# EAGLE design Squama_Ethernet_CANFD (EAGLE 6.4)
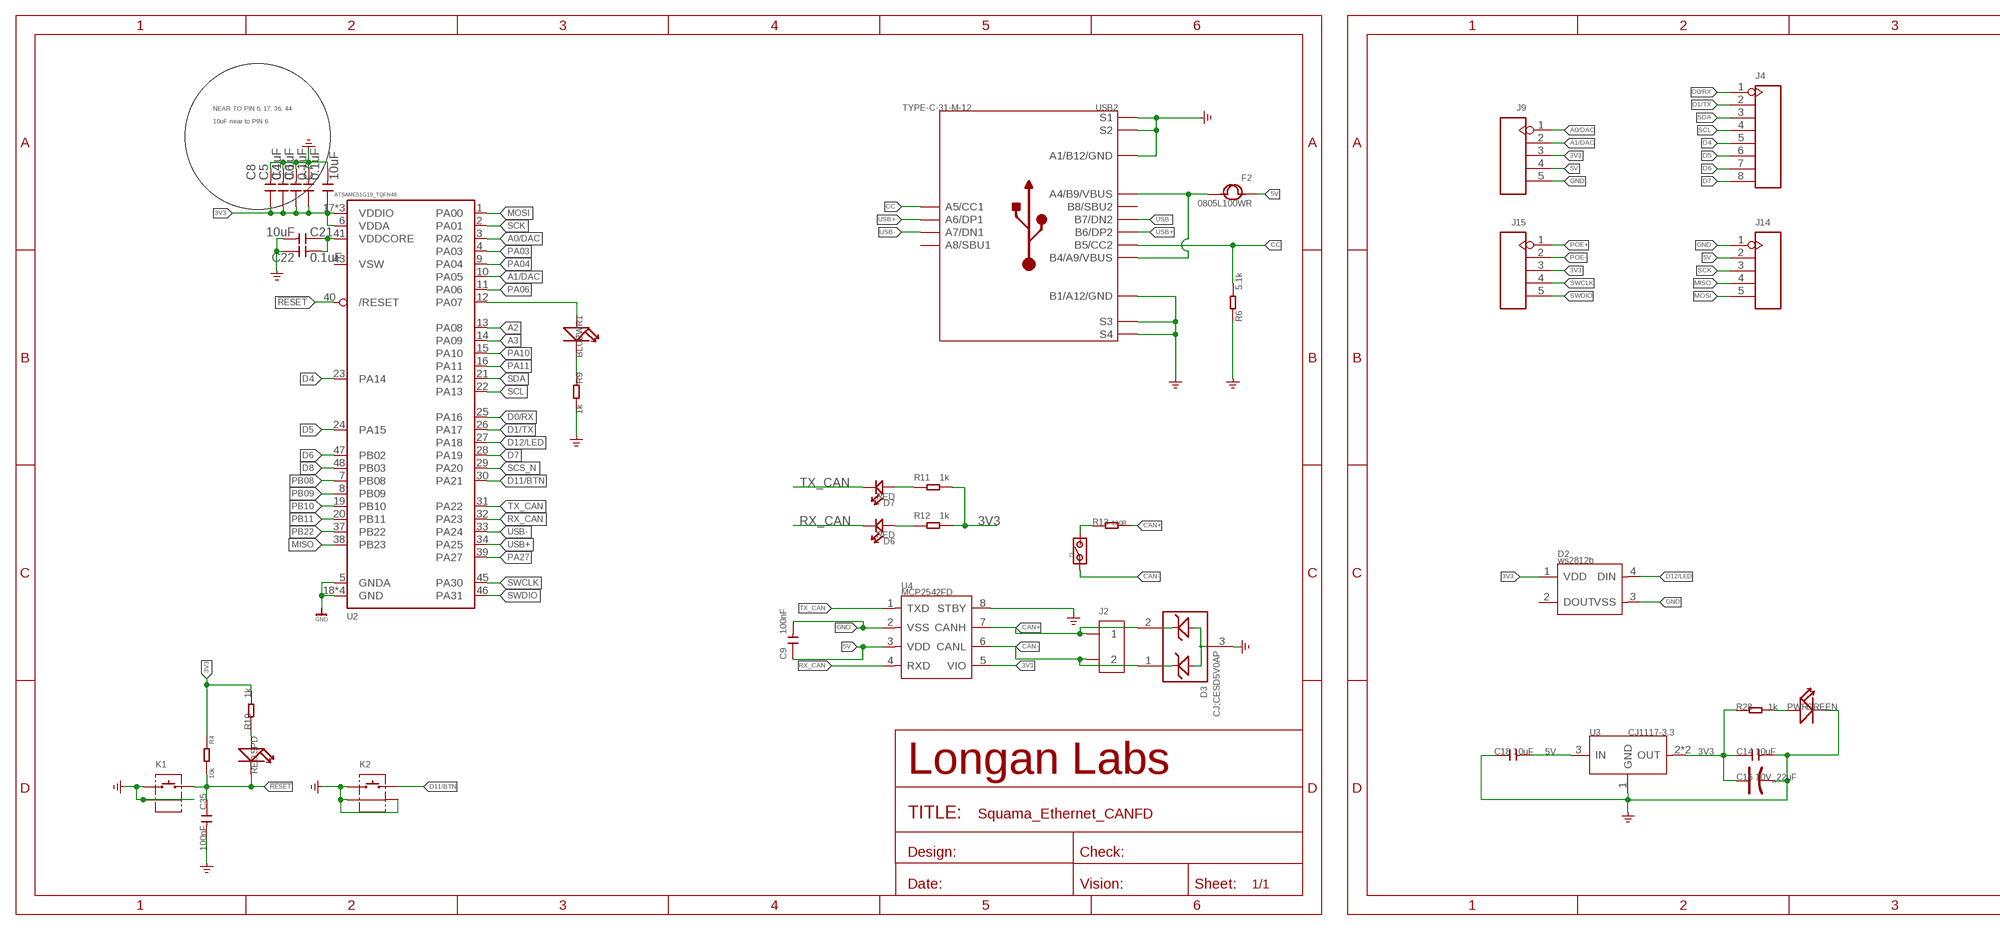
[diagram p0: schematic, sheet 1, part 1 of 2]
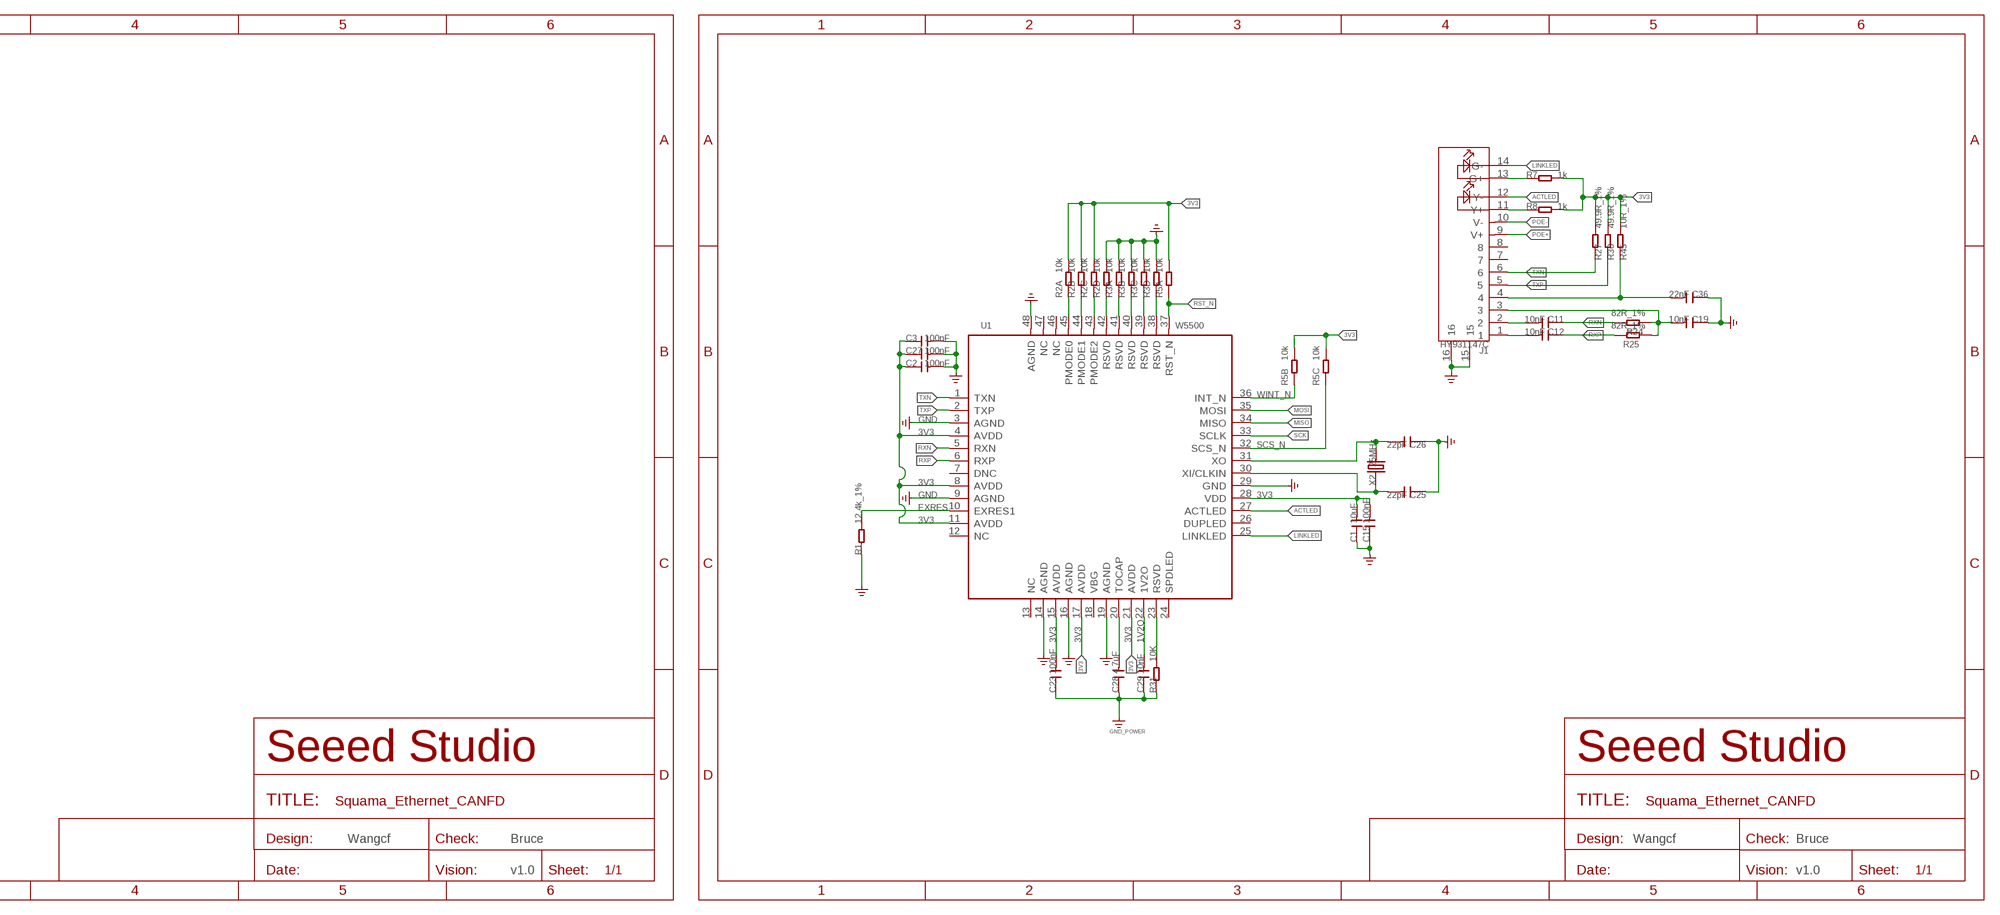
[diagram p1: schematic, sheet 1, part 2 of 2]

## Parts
C1  10uF  C-0603  [C0603]
C2  100nF  C-0603  [C0603]
C3  100nF  C-0603  [C0603]
C4  0.1uF  CAP-0603  [C0603]
C5  0.1uF  CAP-0603  [C0603]
C6  0.1uF  CAP-0603  [C0603]
C7  10uF  CAP-0603  [C0603]
C8  0.1uF  CAP-0603  [C0603]
C9  100nF  CAP-0603  [C0603]
C11  10nF  C-0603  [C0603]
C12  10nF  C-0603  [C0603]
C14  10uF  C-0805  [C0805]
C15  100nF  C-0603  [C0603]
C16  10V_22uF  CAP-AVX-B  [AVX-B]
C18  10uF  C-0805  [C0805]
C19  10nF  C-0603  [C0603]
C21  0.1uF  CAP-0603  [C0603]
C22  10uF  CAP-0603  [C0603]
C23  100nF  C-0603  [C0603]
C25  22pF  C-0603  [C0603]
C26  22pF  C-0603  [C0603]
C27  100nF  C-0603  [C0603]
C28  4.7uF  C-0805  [C0805]
C29  10nF  C-0603  [C0603]
C35  100nF  CAP-0603  [C0603]
C36  22nF  C-0603  [C0603]
D2  ws2812b  LED-RGB-4P-WS2812B-304990003  [LED4-SMD-5050]
D3  CJ;CESD5V0AP  D-ESD-3P'CESD3V3AP'  [SOT-23]
D6  RED  LED'0603'  [LED-0603]
D7  RED  LED'0603'  [LED-0603]
F2  0805L100WR  FUSE0805  [F0805]
J1  HY931147C  RJ45-HY931147C  [RJ45-14+2P-16.1X21.6X13.95MM]
J2  SCREW-TERMINAL-2P'3.5'  [H2-3.5-7.0X7.0MM]
J4  HEADER-8P-80/40MIL  [H8-2.54-C80D40MIL]
J9  HEADER-5P-2.54  [H5-2.54]
J14  HEADER-5P-2.0  [H5-2.0]
J15  HEADER-5P-2.0  [H5-2.0]
K1  BUTTON-2+2P  [SW2+2P-7.7X2.75X3.95MM]
K2  BUTTON-2+2P  [SW2+2P-7.7X2.75X3.95MM]
P1  PAD-JUMPER-2P  [2P-SMD-1.78X1.27]
PWR  GREEN  LED'0603'  [LED-0603]
PWR1  BLUE  LED'0603'  [LED-0603]
R1  12.4k_1%  R-0603  [0603]
R2  10k  RES-ARRAY-0804  [R0804-8]
R3  10k  RES-ARRAY-0804  [R0804-8]
R4  10k  RES-0603  [R0603]
R5  10k  RES-ARRAY-0804  [R0804-8]
R6  5.1k  RES-0603  [R0603]
R7  1k  R-0603  [0603]
R8  1k  R-0603  [0603]
R9  1k  R-0603  [0603]
R10  1k  R-0603  [0603]
R11  1k  RES-0603  [R0603]
R12  1k  RES-0603  [R0603]
R13  120R  R-0603  [0603]
R24  82R_1%  R-0603  [0603]
R25  82R_1%  R-0603  [0603]
R27  49.9R_1%  R-0603  [0603]
R28  1k  R-0603  [0603]
R30  49.9R_1%  R-0603  [0603]
R31  10K  R-0603  [0603]
R45  10R_1%  R-0603  [0603]
SPD  RED  LED'0603'  [LED-0603]
U1  W5500  DRIVER-W5500  [LQFP-48]
U2  ATSAME51G19_TQFN48  [TQFN48_7MM]
U3  CJ1117-3.3  PMIC-CJ1117'SOT89'  [SOT-89]
U4  MCP2542FD  TRANSCEIVER-MCP2542  [SOIC8-1.27-5X4MM]
USB2  TYPE-C-31-M-12  USB2.0-TYPE-C  [USB2.0-TYPE-C]
X2  25MHz  CRYSTAL'5032'  [2P-SMD-5X3.2]

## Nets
1V2O: C29.2 U1.22(1V2O)
3V3: C1.2 C2.1 C3.1 C4.1 C5.1 C6.1 C7.1 C8.1 C14.1 C15.2 C16.+ C23.2 C27.1 D2.1(VDD) J9.3 J15.3 R2.6 R2.7 R2.8 R4.1 R5.6 R5.7 R5.8 R7.2 R8.2 R10.2 R11.2 R12.2 R27.2 R28.1 R30.2 R45.2 U1.4(AVDD) U1.8(AVDD) U1.11(AVDD) U1.15(AVDD) U1.17(AVDD) U1.21(AVDD) U1.28(VDD) U2.6(VDDA) U2.17(VDDIO) U2.36(VDDIO) U2.44(VDDIO) U3.2(OUT) U3.4(OUT) U4.5(VIO)
5V [usbvcc]: C9.1 C18.2 F2.1 J9.4 J14.2 U3.3(IN) U4.3(VDD)
!RESET: C35.1 K1.2 R4.2 SPD.- U2.40(/RESET)
A0/DAC: J9.1 U2.3(PA02)
A1/DAC: J9.2 U2.10(PA05)
A2: U2.13(PA08)
A3: U2.14(PA09)
ACTLED: J1.12(Y-) U1.27(ACTLED)
CAN+: D3.2 J2.1 R13.2 U4.7(CANH)
CAN-: D3.1 J2.2 P1.1 U4.6(CANL)
CC: R6.2 USB2.A5(A5/CC1) USB2.B5(B5/CC2)
D0/RX: J4.1 U2.25(PA16)
D1/TX: J4.2 U2.26(PA17)
D4: J4.5 U2.23(PA14)
D5: J4.6 U2.24(PA15)
D6: J4.7 U2.47(PB02)
D7: J4.8 U2.28(PA19)
D8: U2.48(PB03)
D11/BTN: K2.2 U2.30(PA21)
D12/LED: D2.4(DIN) U2.27(PA18)
EXRES: R1.2 U1.10(EXRES1)
GND: C1.1 C2.2 C3.2 C4.2 C5.2 C6.2 C7.2 C8.2 C9.2 C14.2 C15.1 C16.- C18.1 C19.1 C21.1 C22.2 C23.1 C25.1 C26.1 C27.2 C28.1 C29.1 C35.2 C36.1 D2.3(VSS) D3.3 J1.15 J1.16 J9.5 J14.1 K1.1 K1.S1 K1.S2 K2.1 K2.S1 K2.S2 PWR.- R1.1 R2.5 R3.5 R3.6 R3.7 R3.8 R6.1 R9.2 R31.1 U1.3(AGND) U1.9(AGND) U1.14(AGND) U1.16(AGND) U1.19(AGND) U1.29(GND) U1.48(AGND) U2.5(GNDA) U2.18(GND) U2.35(GND) U2.42(GND) U2.THERMAL(GND) U3.1(GND) U4.2(VSS) U4.8(STBY) USB2.A1_B12(A1/B12/GND) USB2.B1_A12(B1/A12/GND) USB2.S1 USB2.S2 USB2.S3 USB2.S4 USB2.S5(S1) USB2.S6(S2) ; supply symbol labelled GND_POWER
LINKLED: J1.14(G-) U1.25(LINKLED)
MISO: J14.4 U1.34(MISO) U2.38(PB23)
MOSI: J14.5 U1.35(MOSI) U2.1(PA00)
N$1: C25.2 U1.30(XI/CLKIN) X2.1
N$2: PWR1.- R9.1
N$3: F2.2 USB2.A4_B9(A4/B9/VBUS) USB2.B4_A9(B4/A9/VBUS)
N$4: J1.13(G+) R7.1
N$5: J1.11(Y+) R8.1
N$6: R10.1 SPD.+
N$7: PWR1.+ U2.12(PA07)
N$8: D7.+ R11.1
N$9: C21.2 C22.1 U2.41(VDDCORE)
N$10: P1.2 R13.1
N$15: D6.+ R12.1
N$16: C36.2 J1.4 R45.1
N$23: C11.2 J1.2
N$24: C12.2 J1.1
N$26: PWR.+ R28.2
N$27: R3.4 U1.38(RSVD)
N$30: R3.3 U1.39(RSVD)
N$31: R3.2 U1.40(RSVD)
N$32: R3.1 U1.41(RSVD)
N$33: R2.4 U1.42(RSVD)
N$34: C19.2 J1.3 R24.2 R25.1
N$35: R2.3 U1.43(PMODE2)
N$36: R2.2 U1.44(PMODE1)
N$37: R2.1 U1.45(PMODE0)
N$50: R31.2 U1.23(RSVD)
PA03: U2.4(PA03)
PA04: U2.9(PA04)
PA06: U2.11(PA06)
PA10: U2.15(PA10)
PA11: U2.16(PA11)
PA27: U2.39(PA27)
PB08: U2.7(PB08)
PB09: U2.8(PB09)
PB10: U2.19(PB10)
PB11: U2.20(PB11)
PB22: U2.37(PB22)
POE+: J1.9(V+) J15.1
POE-: J1.10(V-) J15.2
RST_N: R5.1 U1.37(RST_N)
RX_CAN: D6.- U2.32(PA23) U4.4(RXD)
RXN: C11.1 R24.1 U1.5(RXN)
RXP: C12.1 R25.2 U1.6(RXP)
SCK: J14.3 U1.33(SCLK) U2.2(PA01)
SCL: J4.4 U2.22(PA13)
SCS_N: R5.3 U1.32(SCS_N) U2.29(PA20)
SDA: J4.3 U2.21(PA12)
SWCLK: J15.4 U2.45(PA30)
SWDIO: J15.5 U2.46(PA31)
TOCAP: C28.2 U1.20(TOCAP)
TX_CAN: D7.- U2.31(PA22) U4.1(TXD)
TXN: J1.6 R27.1 U1.1(TXN)
TXP: J1.5 R30.1 U1.2(TXP)
USB+: U2.34(PA25) USB2.A6(A6/DP1) USB2.B6(B6/DP2)
USB-: U2.33(PA24) USB2.A7(A7/DN1) USB2.B7(B7/DN2)
WINT_N: R5.2 U1.36(INT_N)
XO: C26.2 U1.31(XO) X2.2
Unconnected: D2.2(DOUT) J1.7 J1.8 R5.4 R5.5 U1.7(DNC) U1.12(NC) U1.13(NC) U1.18(VBG) U1.24(SPDLED) U1.26(DUPLED) U1.46(NC) U1.47(NC) U2.43(VSW) USB2.A8(A8/SBU1) USB2.B8(B8/SBU2)

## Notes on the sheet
- NEAR TO PIN 6, 17, 36, 44
- 10uF near to PIN 6
- Wangcf | Bruce | Wangcf | Bruce
- v1.0 | v1.0

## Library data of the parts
C1-C3 C11 C12 C14 C15 C18 C19 C23 C25-C29 C36 = Discrete:C*: Ceramic Capacitors
C4-C9 C21 C22 C35 = Discrete-new:CAP: Ceramic Capacitors
C16 = Discrete:CAP*: Electrolytic Capacitors,Tantalum Capacitors and Super Capacitors
D2 = Discrete-new:LED-RGB-4P
D3 = Discrete-new:D-ESD-3P: 304060003
D6 D7 = Discrete-new:LED
F2 = Discrete-small:FUSE
J1 = Connector-new:RJ45-HY931147C
J2 = Connector-new:SCREW-TERMINAL-2P: 2P-3.5:320110028;2P-5.0:320110031
J4 = Connector-new:HEADER-8P
J9 J14 J15 = Connector-new:HEADER-5P
K1 K2 = Connector-new:BUTTON-2+2P
P1 = Discrete:PAD-JUMPER-2P
PWR PWR1 SPD = Discrete:LED*
R1 R7-R10 R13 R24 R25 R27 R28 R30 R31 R45 = Discrete:R*
R2 R3 R5 = Discrete-new:RES-ARRAY: Resistor Array
R4 R6 R11 R12 = Discrete-new:RES
U1 = template:DRIVER-W5500
U2 = MyLibrary:ATSAME51G19; MPN: ATSAME51G19A-MF
U3 = IC-new:PMIC-CJ*1117: Low Drop Fixed And Adjustable Positive Voltage Regulators http://www.datasheetcatalog.org/datasheet/SGSThomsonMicroelectronics/mXuqtqv.pdf
U4 = untitled:TRANSCEIVER-MCP2542
USB2 = Connector-new:USB2.0-TYPE-C
X2 = Discrete:CRYSTAL*: CRYSTAL

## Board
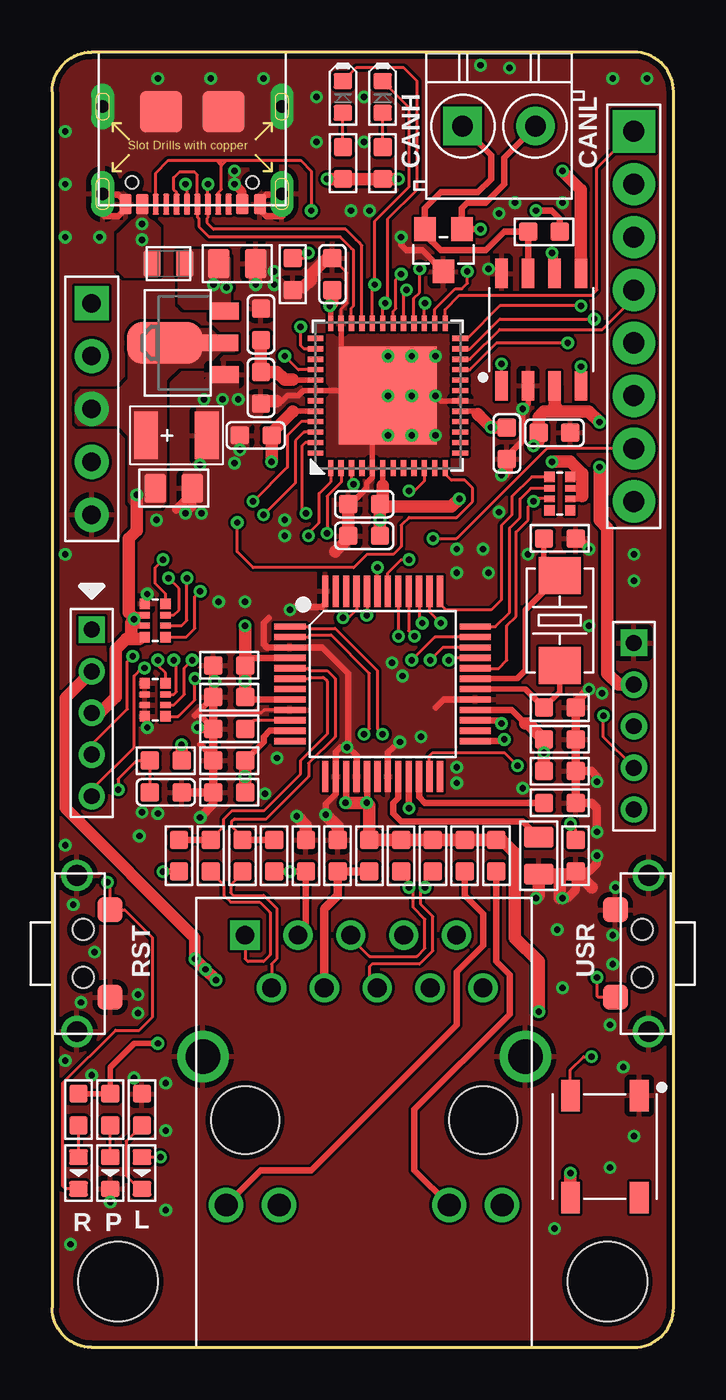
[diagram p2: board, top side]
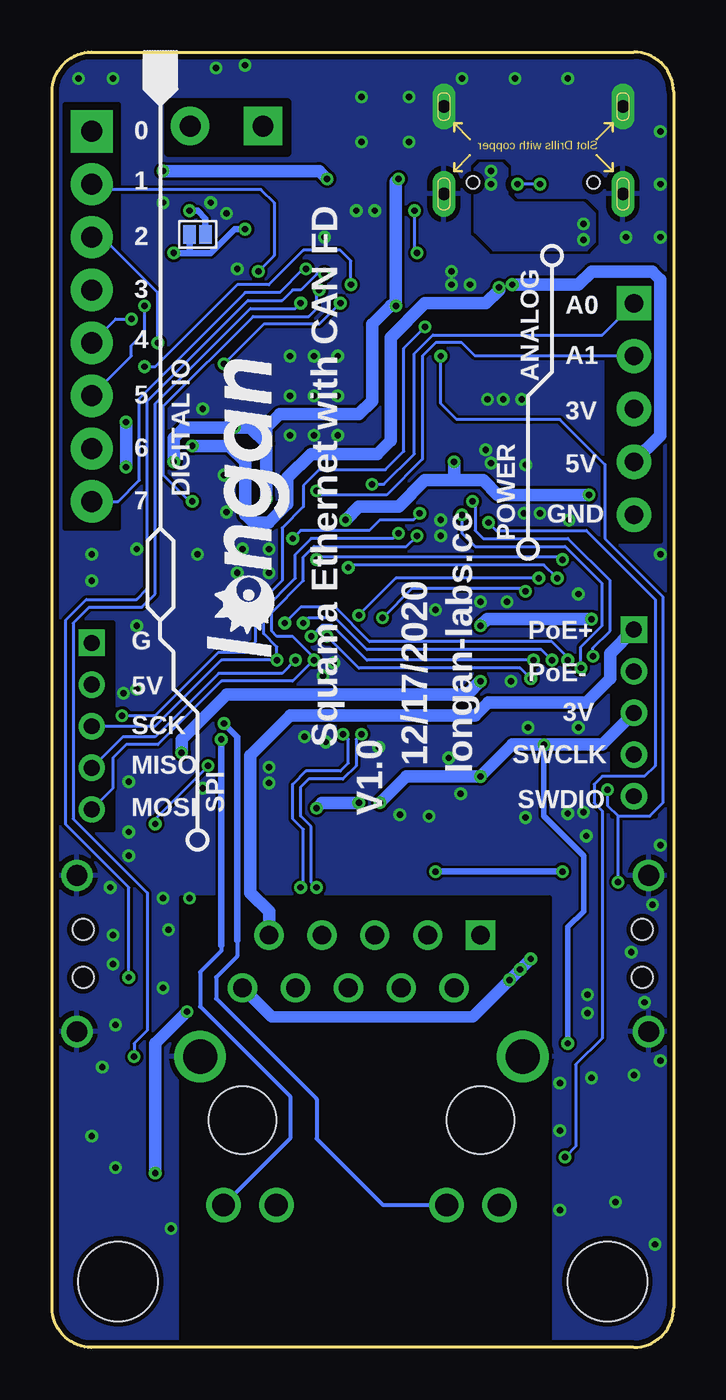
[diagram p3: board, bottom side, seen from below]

Size 29.84 x 62.23 mm. Coordinates in mm from the lower left corner, seen from the top.
Outline: 1.91,0 27.94,0 arc90 29.84,1.91 29.84,60.33 arc90 27.94,62.23 1.91,62.23 arc90 0,60.33 0,1.91 arc90 1.91,0
Copper layers (1*16): Top 0.035mm / dielectric 1.5mm / Bottom 0.035mm
Design rules "default *": minimum track width 5mil, minimum drill 12mil, track to track 4mil, track to pad 4mil, pad to pad 4mil, via to via 4mil, smd to smd 0mil, copper to edge 10mil, drill to drill 10mil, minimum pad ring 10mil, minimum via ring 6mil, stop-mask expansion 2mil, vias tented up to drill 25mil, thermal gap 10mil
Holes 3.81 mm at 26.67,3.17 3.17,3.17
bRestrict: area 0.6,38.7 to 3.2,51.4; area 0.9,25.5 to 2.9,35.4; area 26.7,39.4 to 29.2,59.7; area 26.9,24.9 to 29,34.8; area 6,0 to 23.6,21.6; area 0.6,38.7 to 3.2,51.4; area 18.5,57.4 to 24.3,59.8

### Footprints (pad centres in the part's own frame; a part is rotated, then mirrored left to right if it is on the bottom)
C0603 = smd 0.889 x 0.889: 1 -0.762,0; 2 0.762,0
C0805 = smd 1.016 x 1.397: 1 -0.889,0; 2 0.889,0
AVX-B = smd 1.143 x 2.286: + -1.46,0; - 1.46,0
LED4-SMD-5050 = smd 0.9 x 1.5: 1 -1.65,-2.45; 2 1.65,-2.45; 3 1.65,2.45; 4 -1.65,2.45
SOT-23 = smd 1.016 x 1.143: 1 -0.889,-1.016; 2 0.889,-1.016; 3 0,1.016
LED-0603 = smd 0.762 x 0.889: + 0.762,0; - -0.762,0
F0805 = smd 0.819 x 1.27: 1 -0.79,0; 2 0.79,0
RJ45-14+2P-16.1X21.6X13.95MM = drill 0.9 pad 1.4 square: 1 5.72,-8.89 | drill 0.9 pad 1.4: 2 4.45,-6.35; 3 3.18,-8.89; 4 1.91,-6.35; 5 0.64,-8.89; 6 -0.63,-6.35; 7 -1.9,-8.89; 8 -3.17,-6.35; 9 -4.44,-8.89; 10 -5.71,-6.35 | drill 1.1 pad 1.6: 11 6.625,4.08; 12 4.085,4.08; 13 -4.085,4.08; 14 -6.625,4.08 | drill 1.65 pad 2.3: 15 7.745,-3.05; 16 -7.745,-3.05 | hole 3.25: -5.715,0; 5.715,0
H2-3.5-7.0X7.0MM = drill 1 pad 1.85 square: 1 -1.75,0 | drill 1 pad 1.85: 2 1.75,0
H8-2.54-C80D40MIL = drill 1.016 pad 2.032 square: 1 0,8.89 | drill 1.016 pad 2.032: 2 0,6.35; 3 0,3.81; 4 0,1.27; 5 0,-1.27; 6 0,-3.81; 7 0,-6.35; 8 0,-8.89
H5-2.54 = drill 0.889 pad 1.651 square: 1 0,5.08 | drill 0.889 pad 1.651: 2 0,2.54; 3 0,0; 4 0,-2.54; 5 0,-5.08
H5-2.0 = drill 0.762 pad 1.27 square: 1 0,4 | drill 0.762 pad 1.27: 2 0,2; 3 0,0; 4 0,-2; 5 0,-4
SW2+2P-7.7X2.75X3.95MM = smd 1.2 x 1.2: 1 -2.1,0; 2 2.1,0 | drill 1 pad 1.5: S1 -3.75,1.6; S2 3.75,1.6 | hole 1: -1.15,1.3; 1.15,1.3
2P-SMD-1.78X1.27 = smd 0.889 x 0.61: 1 0,0.381; 2 0,-0.381
LED-0603' = smd 0.762 x 0.889: + -0.762,0; - 0.762,0
0603 = smd 0.889 x 0.889: 1 -0.762,0; 2 0.762,0
R0804-8 = smd 0.498 x 0.5: 1 -0.801,-0.5; 4 0.801,-0.5; 5 0.801,0.5; 8 -0.801,0.5 | smd 0.3 x 0.5: 2 -0.25,-0.5; 3 0.25,-0.5; 6 0.25,0.5; 7 -0.25,0.5
R0603 = smd 0.889 x 0.889: 1 -0.762,0; 2 0.762,0
LQFP-48 = smd 1.5 x 0.3: 1 -4.45,2.75; 2 -4.45,2.25; 3 -4.45,1.75; 4 -4.45,1.25; 5 -4.45,0.75; 6 -4.45,0.25; 7 -4.45,-0.25; 8 -4.45,-0.75; 9 -4.45,-1.25; 10 -4.45,-1.75; 11 -4.45,-2.25; 12 -4.45,-2.75; 25 4.45,-2.75; 26 4.45,-2.25; 27 4.45,-1.75; 28 4.45,-1.25; 29 4.45,-0.75; 30 4.45,-0.25; 31 4.45,0.25; 32 4.45,0.75; 33 4.45,1.25; 34 4.45,1.75; 35 4.45,2.25; 36 4.45,2.75 | smd 0.3 x 1.5: 13 -2.75,-4.45; 14 -2.25,-4.45; 15 -1.75,-4.45; 16 -1.25,-4.45; 17 -0.75,-4.45; 18 -0.25,-4.45; 19 0.25,-4.45; 20 0.75,-4.45; 21 1.25,-4.45; 22 1.75,-4.45; 23 2.25,-4.45; 24 2.75,-4.45; 37 2.75,4.45; 38 2.25,4.45; 39 1.75,4.45; 40 1.25,4.45; 41 0.75,4.45; 42 0.25,4.45; 43 -0.25,4.45; 44 -0.75,4.45; 45 -1.25,4.45; 46 -1.75,4.45; 47 -2.25,4.45; 48 -2.75,4.45
TQFN48_7MM = smd 0.25 x 0.75: 1 -2.75,-3.475; 2 -2.25,-3.475; 3 -1.75,-3.475; 4 -1.25,-3.475; 5 -0.75,-3.475; 6 -0.25,-3.475; 7 0.25,-3.475; 8 0.75,-3.475; 9 1.25,-3.475; 10 1.75,-3.475; 11 2.25,-3.475; 12 2.75,-3.475; 25 2.75,3.475; 26 2.25,3.475; 27 1.75,3.475; 28 1.25,3.475; 29 0.75,3.475; 30 0.25,3.475; 31 -0.25,3.475; 32 -0.75,3.475; 33 -1.25,3.475; 34 -1.75,3.475; 35 -2.25,3.475; 36 -2.75,3.475 | smd 0.75 x 0.25: 13 3.475,-2.75; 14 3.475,-2.25; 15 3.475,-1.75; 16 3.475,-1.25; 17 3.475,-0.75; 18 3.475,-0.25; 19 3.475,0.25; 20 3.475,0.75; 21 3.475,1.25; 22 3.475,1.75; 23 3.475,2.25; 24 3.475,2.75; 37 -3.475,2.75; 38 -3.475,2.25; 39 -3.475,1.75; 40 -3.475,1.25; 41 -3.475,0.75; 42 -3.475,0.25; 43 -3.475,-0.25; 44 -3.475,-0.75; 45 -3.475,-1.25; 46 -3.475,-1.75; 47 -3.475,-2.25; 48 -3.475,-2.75 | smd 4.7 x 4.7: THERMAL 0,0
SOT-89 = smd 0.8 x 1.4: 1 -1.524,-1.905; 3 1.524,-1.905 | smd 0.8 x 1.9: 2 0,-1.651 | smd 2.032 x 3.65: 4 0,0.94
SOIC8-1.27-5X4MM = smd 0.6 x 1.4: 1 -1.905,-2.7; 2 -0.635,-2.7; 3 0.635,-2.7; 4 1.905,-2.7; 5 1.905,2.7; 6 0.635,2.7; 7 -0.635,2.7; 8 -1.905,2.7
USB2.0-TYPE-C = smd 1 x 0.6: A1_B12 -0.05,3.25; A4_B9 -0.05,2.4; B1_A12 -0.05,-3.2; B4_A9 -0.05,-2.4 | smd 1 x 0.3: A5 -0.05,1.25; A6 -0.05,0.25; A7 -0.05,-0.25; A8 -0.05,-1.25; B5 -0.05,-1.75; B6 -0.05,-0.75; B7 -0.05,0.75; B8 -0.05,1.75 | drill 0.6 pad 1 long: S1 -4.75,4.3; S2 -4.75,-4.3 | drill 0.6 pad 1.1 long: S3 -0.55,4.3; S4 -0.55,-4.3 | smd 2 x 2: S5 -4.5,1.5; S6 -4.5,-1.5 | hole 0.6: -1.1,-2.89; -1.1,2.89
2P-SMD-5X3.2 = smd 1.778 x 2.032: 1 -2.159,0; 2 2.159,0

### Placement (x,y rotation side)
C1  24.38,27.69 180 top
C2  8.51,28.19 180 top
C3  8.51,32.77 180 top
C4  13.46,51.56 90 top
C5  9.78,43.81 180 top
C6  21.84,43.43 270 top
C7  14.99,38.99 180 top
C8  14.99,40.51 180 top
C9  24.13,43.94 0 top
C11  9.14,23.62 270 top
C12  7.62,23.62 270 top
C14  5.84,41.27 0 top
C15  24.38,29.21 180 top
C16  5.97,43.81 0 top
C18  8.89,52.07 180 top
C19  12.19,23.62 270 top
C21  10.03,49.15 270 top
C22  10.03,46.1 270 top
C23  8.51,26.67 0 top
C25  24.38,30.73 180 top
C26  24.38,38.86 180 top
C27  8.51,31.24 180 top
C28  23.37,23.62 90 top
C29  24.38,26.16 180 top
C35  5.46,26.67 0 top
C36  13.72,23.62 270 top
D2  26.54,9.65 0 top
D3  18.8,52.7 180 top
D6  15.88,60.07 270 top
D7  13.97,60.07 270 top
F2  5.59,52.07 180 top
J1  14.99,10.92 180 top
J2  21.46,58.67 0 top
J4  27.94,49.53 0 top
J9  1.91,45.09 0 top
J14  27.94,29.84 0 top
J15  1.91,30.48 0 top
K1  2.79,18.92 90 top
K2  27.05,18.92 270 top
P1  22.86,53.47 90 bottom
PWR  GREEN  [LED-0603']  2.79,8.38 270 top
PWR1  BLUE  [LED-0603']  4.32,8.38 270 top
R1  8.51,29.72 0 top
R2  4.95,34.92 90 top
R3  4.95,31.11 90 top
R4  5.46,28.19 180 top
R5  24.38,41.02 270 top
R6  11.56,51.56 90 top
R7  21.34,23.62 90 top
R8  19.81,23.62 90 top
R9  4.32,11.43 90 top
R10  1.27,11.43 90 top
R11  13.97,56.9 270 top
R12  15.88,56.9 270 top
R13  23.62,53.59 180 top
R24  10.67,23.62 270 top
R25  6.1,23.62 90 top
R27  18.29,23.62 90 top
R28  2.79,11.43 270 top
R30  16.76,23.62 90 top
R31  25.15,23.62 90 top
R45  15.24,23.62 90 top
SPD  RED  [LED-0603']  1.27,8.38 270 top
U1  15.88,31.88 0 top
U2  16.13,45.72 0 top
U3  6.35,48.26 90 top
U4  23.5,48.9 0 top
U$7  [LONGAN-SILK-SMALLER]  17.27,31.88 90 bottom
USB2  6.73,54.86 270 top
X2  24.38,34.92 90 top

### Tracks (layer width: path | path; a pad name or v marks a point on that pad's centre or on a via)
1V2O
  Top 0.305: U1.22 17.62,26.44 17.91,26.16 C29.2
3V3  (via drill 0.3 pad 0.51, 0.3 pad 0.61)
  Top 0.254: R10.2 2.67,12.19 2.79,12.06 R28.1 2.79,13.46 3.94,14.61 v5.08,14.61 | U2.36 13.38,49.99 v13.34,50.04 | U2.6 15.88,41.41 15.88,41.4 | U2.44 11.57,44.97 11.56,44.96 | U2.17 20.31,44.97 20.51,44.77
  Top 0.305: U1.15 14.12,26.19 v14.1,26.16 | U1.17 15.12,26.17 v15.11,26.16 | U1.21 17.12,25.93 v17.14,25.91 | U1.28 22.08,30.63 22.73,29.97 | U1.8 9.39,31.13 C27.1 | U1.11 10.45,29.63 10.16,29.34 10.16,29.08 C2.1 | U1.4 9.63,33.13 C3.1 | R2.7 4.12,34.67 3.94,34.86 3.94,34.92 v3.94,34.99 4.12,35.17 R2.6 | R5.7 25.46,41.27 | R5.6 25.34,40.77 25.46,40.89 | R5.8 25.42,41.82 25.46,41.78
  Top 0.406: R2.8 4.28,34.12 4.19,34.04
  Top 0.61: C23.2 v9.27,27.43 C2.1 | v14.1,26.16 v15.11,26.16 15.24,26.04 R45.2 R30.2 R27.2 R8.2 R7.2 21.59,24.38 22.23,23.75 22.23,19.68 23.37,18.54 v23.37,16.13 | 22.73,29.97 22.86,29.97 C15.2 v23.62,28.57 C1.2 | C27.1 v9.27,32 C3.1 v9.27,34.67 | R4.1 v6.22,28.96 | J15.3 2.29,30.48 3.05,31.24 3.05,33.53 3.56,34.04 3.81,34.04 | 3.81,34.04 4.19,34.04 | 3.81,34.04 3.81,34.8 3.94,34.92 | v3.94,34.99 3.94,35.05 3.68,35.31 3.68,38.86 4.06,39.24 v4.06,40.96 | 25.46,40.89 25.46,41.27 25.46,41.78 25.46,41.97 24.89,42.55 v24,42.55 | D2.1 v24.89,8.38 | C4.1 13.46,50.16 v13.34,50.04 | 15.88,41.4 15.88,40.64 C8.1 15.75,40.39 | 15.75,40.39 v15.75,39.75 C7.1 | v10.54,42.55 C5.1 10.54,43.94 11.56,44.96 | C6.1 v21.08,44.2 20.51,44.77 20.45,44.83 | 15.75,40.39 19.18,40.39 v19.56,40.77 | v13.21,56.13 R11.2 R12.2 v16.64,56.13 | U4.5 25.4,55.63 v24.51,56.52
  Bottom 0.254: v5.08,14.61 5.08,20.19 4.32,20.95 4.32,23.62 6.22,25.53 v6.22,28.96
  Bottom 0.61: v14.1,26.16 12.83,27.43 v9.27,27.43 7.75,28.96 v6.22,28.96 3.43,28.96 J15.3 | v15.11,26.16 16.89,26.16 v17.14,25.91 | v23.62,28.57 C15.2 21.46,31.37 9.91,31.37 v9.27,32 | v3.94,34.99 8.95,34.99 v9.27,34.67 | v24.89,8.38 24.89,14.61 v23.37,16.13 | v4.06,40.96 8.45,40.96 9.14,41.66 10.41,41.66 | v15.75,39.75 15.11,40.39 13.21,40.39 11.94,41.66 10.41,41.66 | v10.54,42.55 10.54,41.78 10.41,41.66 | v24,42.55 24,43.69 23.5,44.2 v21.08,44.2 20.32,44.2 | v19.56,40.77 19.56,43.43 | 19.56,43.43 19.56,44.2 | 20.32,44.2 19.56,44.2 | 19.56,43.43 20.32,44.2 | v13.21,56.13 13.34,56.01 v13.34,50.04 13.59,50.04 14.48,49.15 14.48,45.47 15.11,44.83 18.92,44.83 19.56,44.2 | v24.51,56.52 17.02,56.52 v16.64,56.13
  pour Top (isolate 0.254, no thermals): 7.62,48.9 4.19,48.9 3.68,48.39 3.68,46.48 3.17,45.97 1.4,45.97 1.14,45.72 1.14,44.45 1.27,44.32 3.17,44.32 3.68,43.81 3.68,40.64 3.94,40.39 5.21,40.39 5.46,40.64 5.46,46.48 6.1,47.12 7.37,47.12 8.13,47.88 8.76,47.88 8.76,48.51 8,48.51
5V  (via drill 0.3 pad 0.61)
  Top 0.61: J14.2 27.21,31.84 26.67,32.38 26.67,39.37 26.29,39.75 v26.29,42.29 | U4.3 24.13,45.21 | 24.13,45.21 23.88,44.96 | 24.38,44.96 24.13,44.96 23.88,44.96 | 24.13,45.21 24.38,44.96 | 23.88,44.96 23.62,44.96 23.37,44.7 C9.1 23.37,43.56 v23.11,43.31 | 24.38,44.96 25.78,44.96 v26.29,44.45
  Bottom 0.61: v7.75,51.05 4.57,51.05 3.94,51.69 1.02,51.69 0.64,51.31 0.64,43.81 J9.4 | v8.38,50.93 8.38,50.8 9.02,50.16 11.94,50.16 13.59,48.51 13.59,43.56 14.22,42.93 17.4,42.93 18.54,41.78 18.54,40.51 19.43,39.62 20.19,39.62 20.57,40.01 20.57,42.55 21.34,43.31 v23.11,43.31 | v26.29,42.29 v26.29,44.45
  pour Top (isolate 0.254, no thermals): 6.35,52.7 8,52.7 8.51,52.32 8.51,49.53 8.26,49.53 7.87,49.91 6.35,49.91 6.1,50.16 6.1,52.45
!RESET  (via drill 0.3 pad 0.61)
  Top 0.152: C35.1 R4.2 4.06,28.19 3.17,27.3 v3.17,26.8 | SPD.- 0.64,7.62 0.51,7.75 0.51,12.7 3.05,15.24 4.19,15.24 4.83,15.88 4.83,19.68 3.49,21.02 K1.2 2.79,22.23 v2.67,22.35 | U2.40 11.83,46.97 v11.18,47.62
  Bottom 0.152: v3.17,26.8 3.17,26.04 2.67,25.53 | 2.67,25.53 1.14,25.53 0.51,26.16 0.51,36.07 3.3,38.86 3.3,42.42 5.46,44.58 10.41,44.58 11.18,45.34 v11.18,47.62 | v2.67,22.35 2.67,25.53
A0/DAC  (via drill 0.3 pad 0.61)
  Top 0.152: U2.3 14.38,41.56 v14.48,41.47
  Bottom 0.152: v14.48,41.47 13.91,41.47 12.45,42.93 12.45,47.75 11.56,48.64 3.43,48.64 J9.1
A1/DAC  (via drill 0.3 pad 0.61)
  Top 0.152: U2.10 17.88,41.63 17.4,41.15 v17.14,41.15
  Bottom 0.152: J9.2 9.53,47.62 10.16,48.26 11.43,48.26 12.06,47.62 12.06,42.67 13.78,40.96 16.95,40.96 v17.14,41.15
ACTLED  (via drill 0.3 pad 0.61)
  Top 0.305: U1.27 21.43,30.13 v21.59,29.97
  Bottom 0.203: 20.95,19.56 20.95,18.8 21.97,17.78 21.97,16.76 17.14,11.94 17.14,10.03 13.97,6.86 10.92,6.86 J1.12
  Bottom 0.305: 20.95,19.56 20.95,29.34 v21.59,29.97
CAN+
  Top 0.305: U4.7 R13.2 21.72,53.59 20.83,52.7 18.67,52.7 17.91,53.47 D3.2 17.91,54.74 18.67,55.5 20.45,55.5 21.08,56.13 21.08,57.28 19.71,58.65 J2.1
CAN-  (via drill 0.3 pad 0.51)
  Top 0.305: U4.6 24.13,52.45 v24,52.58 | v20.57,53.72 D3.1 19.68,54.74 19.94,54.99 20.83,54.99 21.72,55.88 21.72,57.15 23.21,58.65 J2.2
  Bottom 0.305: v20.57,53.72 21.08,53.72 22.23,52.58 23.24,52.58 | 23.24,52.58 v24,52.58 | P1.1 23.24,52.58
CC  (via drill 0.3 pad 0.61)
  Top 0.152: USB2.A5 7.98,55.48 8.13,55.63 8.13,56.77 | USB2.B5 4.98,56.42 5.59,57.02 7.87,57.02 | 8.13,56.77 8.13,57.02 | 7.87,57.02 8.13,57.02 | 8.13,57.02 8.38,57.02 | 8.38,57.02 11.94,57.02 12.45,56.52 v12.45,54.61 | 8.13,56.77 7.87,57.02 | 8.38,57.02 8.13,56.77 | R6.2 12.06,52.32 v12.32,52.58
  Bottom 0.152: v12.45,54.61 12.45,52.7 v12.32,52.58
D0/RX
  Top 0.152: U2.25 18.88,49.87 19.56,50.55 25.91,50.55 26.16,50.8 26.16,56.64 J4.1
D1/TX  (via drill 0.3 pad 0.51)
  Top 0.152: U2.26 18.38,49.88 19.37,50.86 19.68,50.86 19.94,51.12 v19.94,51.69
  Bottom 0.152: J4.2 27.69,55.63 19.81,55.63 19.18,54.99 19.18,52.45 v19.94,51.69
D4  (via drill 0.3 pad 0.61)
  Top 0.152: U2.23 20.07,47.97 21.5,49.4 v26.04,49.4
  Bottom 0.152: J4.5 26.8,49.4 v26.04,49.4
D5  (via drill 0.3 pad 0.61)
  Top 0.152: U2.24 19.94,48.47 21.51,50.04 v25.4,50.04
  Bottom 0.152: J4.6 26.04,47.62 26.04,48.13 25.4,48.77 v25.4,50.04
D6  (via drill 0.3 pad 0.61)
  Top 0.152: U2.47 12.16,43.47 12,43.31 12,40.26 v12.19,40.07 | J4.7 23.75,43.18 19.43,38.86 v18.29,38.86
  Bottom 0.152: v12.19,40.07 12.51,39.75 14.1,39.75 14.61,39.24 17.91,39.24 v18.29,38.86
D7  (via drill 0.3 pad 0.51)
  Top 0.152: U2.28 17.38,50.4 17.65,50.67 v17.65,51.82
  Bottom 0.152: J4.8 26.67,40.64 25.65,41.66 25.65,45.59 20.57,50.67 18.92,50.67 17.78,51.82 v17.65,51.82
D11/BTN  (via drill 0.3 pad 0.51, 0.3 pad 0.61)
  Top 0.152: K2.2 26.22,16.82 26.16,16.88 v26.16,17.78 | U2.30 16.38,49.78 16.51,49.91 16.51,51.31 v16.76,51.56
  Bottom 0.152: v26.16,17.78 26.16,22.1 29.21,25.15 29.21,34.92 28.19,35.94 25.78,35.94 25.27,36.45 25.27,45.47 20.45,50.29 18.8,50.29 18.29,50.8 17.91,50.8 17.14,51.56 v16.76,51.56
D12/LED  (via drill 0.3 pad 0.51, 0.3 pad 0.61)
  Top 0.152: D2.4 24.89,13.34 25.53,13.97 v25.91,13.97 | U2.27 17.88,50.14 v17.91,50.16
  Bottom 0.152: v25.91,13.97 25.91,14.61 25.27,15.24 25.27,21.84 28.83,25.4 28.83,34.8 28.07,35.56 25.53,35.56 24.89,36.2 24.89,45.34 20.32,49.91 18.16,49.91 v17.91,50.16
EXRES
  Top 0.152: U1.10 9.68,30.13 R1.2
GND  (via drill 0.3 pad 0.61)
  Top 0.152: U1.9 10.18,30.63 10.03,30.48 7.75,30.48 | U2.35 13.88,49.88 14.16,50.16 14.16,51.63 C4.2
  Top 0.254: C8.2 14.35,40.51 15.11,41.27 15.11,41.53 15.38,41.8 U2.5 15.38,43.83 15.62,44.07 | U4.2 22.86,45.34 v22.61,45.09 22.61,43.56 21.84,42.8 C6.2 | 10.79,45.47 11.05,45.47 11.3,45.72 11.81,45.72 12.06,45.97 U2.42 14.98,45.97 14.99,45.97 | U2.18 18.66,45.47 v18.41,45.72 | U2.35 13.88,47.97 14.22,47.62
  Top 0.305: C27.2 6.86,30.35 | R1.1 7.11,30.35 | C2.2 7.75,28.32 7.11,28.96 | 2.54,54.36 3.17,54.36 3.53,54.71 USB2.B1_A12 3.53,55.02 3.17,55.37 2.41,55.37 2.43,55.39 USB2.S4 | 11.05,54.36 10.29,54.36 9.98,54.66 USB2.A1_B12 9.98,55.07 10.29,55.37 10.99,55.37 USB2.S3 | 10.41,35.05 10.16,34.8 10.16,33.78 10.31,33.63 U1.3 12.98,33.63 14.22,32.38 14.22,28.89 v14.16,28.83 13.84,28.83 13.62,28.61 U1.14 13.62,26.58 13.14,26.1 v13.14,25.59 | U1.16 14.62,28.43 14.22,28.83 | U1.19 16.12,28.57 16.38,28.83 | U1.29 18.81,31.13 18.41,30.73 | U1.48 13.12,35.73 12.95,35.56 11.56,35.56 v11.43,35.43 | D3.3 17.78,52.7 17.02,52.7 16.76,52.96 v16.76,53.34
  Top 0.406: 6.35,40.01 v6.41,40.07 6.73,40.39 C14.2 6.73,41.02 5.97,40.26 | C3.2 7.75,32.07 7.78,32.04 | 7.78,32.04 v7.81,32 | 7.78,32.04 7.75,32 C27.2 R1.1 | R1.1 6.99,29.72 | R1.1 C2.2 C23.1 | C35.2 C23.1 | C23.1 7.75,26.1 v7.11,25.46 | C26.1 25.27,38.86 v25.78,38.35 | v25.78,31.62 25.15,30.99 C25.1 C15.1 C1.1 | C1.1 C29.1 25.91,26.16 26.16,25.91 v26.16,24.77 | C1.1 25.91,27.69 26.16,27.43 v26.16,27.18 | v26.16,23.62 26.16,23.24 25.78,22.86 R31.1 25.15,21.97 24.77,21.59 v24.51,21.59
  Top 0.61: C18.1 v9.78,51.05 | C36.1 13.72,25.02 v13.14,25.59 | C19.1 12.19,25.08 v11.75,25.53 | v23.24,21.59 23.37,21.72 C28.1 24.38,22.73 | 24.38,22.73 25.02,22.73 R31.1 25.91,22.1 | 24.38,22.73 24.38,21.59 | C4.2 13.21,52.32 12.45,51.56 12.45,51.31 12.06,50.93 | 10.79,45.47 10.16,45.47 C22.2 | C6.2 21.84,42.16 v21.59,41.91 | C8.2 C7.2 14.22,38.86 13.59,38.23
  other vias: 10.67,51.05 7.29,45.54 25.78,34.67 26.42,31.43 24.26,20.07 24.51,17.27 27.43,13.46 16.7,29.08 6.99,29.78 4.57,29.78 4.57,36.2 0.64,58.42 0.64,55.88 0.64,53.34 0.64,38.1 0.64,24.13 0.64,13.78 27.94,10.16 27.94,38.1 28.57,60.96 7.62,60.96 5.08,60.96 10.16,60.96 5.08,25.65 10.79,28.32 16.83,32.26 2.79,6.99 5.46,6.6 3.94,12.95 24.13,5.71 10.22,26.61 17.72,29.34 8.18,45.54 21.97,61.47 20.57,61.59 2.29,53.34 7.1,42.41 26.92,60.96 16.32,32.89 0.89,4.95 1.4,16.57 2.03,18.99 1.02,21.27 4.32,25.72 26.8,15.49 26.92,18.41 26.92,19.81 27.05,22.1 26.8,8.64 16.13,45.72 17.27,45.72 16.13,47.62 17.27,47.62 18.41,47.62 17.27,43.81 16.13,43.81 18.41,43.81 14.35,54.61 15.24,54.61 20.95,51.82 21.46,54.48 11.18,39.75 11.18,38.99 9.02,43.12 8.76,42.48 14.99,57.91 14.99,60.07 12.7,57.91 12.7,60.07 19.43,38.35 20.7,38.35 20.95,37.21 19.43,37.21 21.46,40.13 8,35.81 9.27,35.81 27.94,36.83 19.43,27.88 19.43,27.11 22.61,26.86 22.86,38.1 22.23,54.99 24.51,54.99 5.46,10.41 5.46,12.7 1.91,13.08 4.13,16.07 4.13,16.95 4.19,24.57 7.18,40.07 5.02,39.75 8.94,45.54 10.67,51.69
  pour Top (isolate 0.127, rank 6): 0,62.23 29.84,62.23 29.84,0 0,0
  pour Bottom (isolate 0.127, rank 6): 0,62.23 29.84,62.23 29.84,0 0,0
  pour Top (isolate 0.254, no thermals): 9.65,52.7 10.54,52.7 10.79,52.45 10.79,51.56 11.18,51.18 12.11,51.18 12.37,50.92 12.37,50.08 11.81,49.53 10.16,49.53 9.53,50.16 9.53,52.58
  pour Top (isolate 0.254, no thermals): 6.35,41.66 6.35,42.04 6.99,42.67 6.99,46.1 7.62,46.74 8.64,46.74 8.89,46.48 8.89,45.97 9.14,45.72 10.03,45.72 10.29,45.47 10.29,45.09 9.4,44.2 9.4,41.53 8.64,40.77 7.62,39.75 6.6,39.75 6.35,40.01
LINKLED  (via drill 0.3 pad 0.61)
  Top 0.305: U1.25 21.63,29.13 v21.72,29.21
  Bottom 0.203: 21.72,19.3 21.72,19.05 22.73,18.03 22.73,16.38 18.41,12.06 18.41,10.04 J1.14
  Bottom 0.305: v21.72,29.21 21.72,19.3
MISO  (via drill 0.3 pad 0.61)
  Top 0.152: U1.34 18.77,33.63 v18.16,33.02 | J14.4 27.94,27.88 26.48,29.34 v26.48,30.35 | U2.38 12.1,47.97 11.94,48.13 v11.94,49.02
  Bottom 0.152: v18.16,33.02 18.8,32.38 21.84,32.38 24.89,29.34 26.45,29.34 J14.4 | v26.48,30.35 24.89,30.35 21.84,33.4 20.57,33.4 20.07,33.91 20.07,35.56 18.8,36.83 18.8,39.37 17.78,40.39 17.78,41.4 17.02,42.16 13.84,42.16 12.95,43.05 12.95,48.01 v11.94,49.02
MOSI  (via drill 0.3 pad 0.61)
  Top 0.152: U1.35 18.38,34.13 v17.27,33.02 | v12.32,38.99 12.32,39.12 12.83,39.62 12.83,41.02 13.38,41.57 U2.1
  Bottom 0.152: J14.5 26.92,26.86 26.92,28.32 26.29,28.96 24.77,28.96 21.72,32 18.29,32 v17.27,33.02 17.27,33.15 18.29,34.16 19.05,34.16 19.3,34.42 19.3,35.31 17.78,36.83 17.78,37.97 17.27,38.48 12.83,38.48 v12.32,38.99
N$1
  Top 0.254: U1.30 22.73,31.63 C25.2 24.38,31.5 X2.1
N$2
  Top 0.152: R9.1 3.56,9.91 3.56,8.26 4.19,7.62 PWR1.-
N$3  (via drill 0.3 pad 0.61)
  Top 0.406: USB2.A4_B9 9.13,55.51 v8.76,55.88
  other vias: 8.76,56.52 4.32,53.98 4.32,53.21
  pour Top (isolate 0.254, no thermals): 8.89,55.12 8.89,55.37 8.51,55.75 8.51,56.64 8.64,56.77 9.27,56.77 9.4,56.64 9.4,55.5 9.27,55.37 9.27,54.74 9.14,54.61 9.02,54.61 8.89,54.74
  pour Bottom (isolate 0.254, no thermals): 9.27,56.9 8.26,56.9 8,56.64 8,55.37 7.62,54.99 4.32,54.99 3.81,54.48 3.81,53.09 4.19,52.7 8.64,52.7 9.53,53.59 9.53,56.64
  pour Top (isolate 0.254, no thermals): 4.32,55.05 4.45,55.05 4.51,54.99 4.51,54.42 5.14,53.78 5.14,51.56 5.02,51.44 3.49,51.44 3.17,51.75 3.17,53.47 4.13,54.42 4.13,54.86
N$4
  Top 0.305: R7.1 21.34,18.54 21.97,17.91 21.97,16 17.4,11.43 17.4,8.51 J1.13
N$5
  Top 0.305: R8.1 19.81,21.72 20.7,20.83 20.7,19.3 19.43,18.03 19.43,15.49 12.45,8.51 10.03,8.51 J1.11
N$6
  Top 0.152: SPD.+ R10.1
N$7  (via drill 0.3 pad 0.51, 0.3 pad 0.61)
  Top 0.152: v8.89,39.62 8.89,38.23 9.65,37.47 14.48,37.47 15.11,38.1 16.38,38.1 16.76,38.48 16.76,39.5 17.14,39.88 19.43,39.88 20.19,40.64 20.19,41.27 19.81,41.66 19.18,41.66 18.88,41.95 U2.12 | v5.21,9.14 PWR1.+
  Bottom 0.152: v8.89,39.62 8.51,39.24 4.19,39.24 0.89,35.94 0.89,27.94 1.4,27.43 3.43,27.43 3.81,27.05 3.81,26.16 3.43,25.78 3.43,14.86 4.7,13.59 4.7,9.65 v5.21,9.14
N$8
  Top 0.152: R11.1 D7.+
N$9
  Top 0.254: U2.41 11.57,46.47 11.56,46.48
  Top 0.61: C21.2 9.91,48.39 10.03,48.26 C22.1 10.79,46.86 11.18,46.48 11.56,46.48
N$10  (via drill 0.3 pad 0.51)
  Top 0.305: v23.24,54.61 24,54.61 24.38,54.23 R13.1
  Bottom 0.305: v23.24,54.61 22.86,54.61 22.48,54.23 P1.2
N$15
  Top 0.152: R12.1 D6.+
N$16
  Top 0.406: J1.4 13.08,21.08 13.72,21.72 C36.2 R45.1
N$23
  Top 0.152: C11.2 9.14,22.8 8.57,22.23 8.57,21.84 8.7,21.72 10.16,21.72 10.79,21.08 10.79,18.67 10.54,18.41 J1.2
N$24
  Top 0.152: C12.2 8.26,22.23 8.26,21.72 8.57,21.4 9.97,21.4 10.48,20.89 10.48,18.86 10.16,18.54 9.4,18.54 9.27,18.67 J1.1
N$26
  Top 0.152: PWR.+ R28.2
N$27  (via drill 0.3 pad 0.61)
  Top 0.152: R3.4 5.45,32.39 5.08,32.77 v5.08,33.02 | U1.38 18.12,35.34 v18.67,34.8
  Bottom 0.152: v5.08,33.02 5.08,33.15 5.84,33.91 14.61,33.91 16.26,35.56 17.91,35.56 v18.67,34.8
N$30  (via drill 0.3 pad 0.61)
  Top 0.152: R3.3 5.84,31.36 5.97,31.5 5.97,32.89 v5.84,33.02 | U1.39 17.62,34.95 v17.78,34.8
  Bottom 0.152: v5.84,33.02 6.35,33.53 14.73,33.53 16.26,35.05 17.53,35.05 v17.78,34.8
N$31  (via drill 0.3 pad 0.61)
  Top 0.152: R3.2 5.85,30.86 6.35,31.37 6.35,32.64 v6.73,33.02 | U1.40 17.12,34.44 v17.4,34.16
  Bottom 0.152: v6.73,33.02 14.73,33.02 16.38,34.67 16.89,34.67 v17.4,34.16
N$32  (via drill 0.3 pad 0.61)
  Top 0.152: R3.1 6.06,30.31 6.86,31.11 v6.86,32.13 | U1.41 16.62,34.17 v16.64,34.16
  Bottom 0.152: v6.86,32.13 7.37,32.64 15.11,32.64 v16.64,34.16
N$33  (via drill 0.3 pad 0.61)
  Top 0.152: R2.4 5.45,36.2 4.95,36.7 4.95,37.47 v5.33,37.85 | U1.42 16.12,37.21 16.76,37.85 v17.14,37.85
  Bottom 0.152: v5.33,37.85 5.46,37.97 17.02,37.97 v17.14,37.85
N$34  (via drill 0.3 pad 0.61)
  Top 0.305: R24.2 v11.43,22.86 C19.2 12.19,20.2 J1.3 | v5.33,22.86 R25.1
  Bottom 0.305: v11.43,22.86 v5.33,22.86
N$35  (via drill 0.3 pad 0.61)
  Top 0.152: R2.3 5.84,35.17 6.1,35.43 6.1,36.45 v5.59,36.96 | U1.43 v15.62,37.46 v15.62,37.47
  Bottom 0.152: v5.59,36.96 6.22,37.59 15.49,37.59 v15.62,37.47
N$36  (via drill 0.3 pad 0.61)
  Top 0.152: R2.2 6.23,34.67 6.48,34.92 v6.48,36.96 | U1.44 15.12,35.19 v15.11,35.18
  Bottom 0.152: v6.48,36.96 13.34,36.96 v15.11,35.18
N$37  (via drill 0.3 pad 0.61)
  Top 0.152: R2.1 6.44,34.12 6.86,34.54 6.86,36.07 v7.11,36.32 | U1.45 14.62,35.45 14.22,35.05 v13.97,35.05
  Bottom 0.152: v7.11,36.32 7.24,36.32 7.37,36.45 12.57,36.45 v13.97,35.05
N$50  (via drill 0.3 pad 0.61)
  Top 0.152: U1.23 18.12,28.41 18.29,28.57 21.72,28.57 v22.35,27.94 | R31.2 25.15,24.89 v24.89,25.15
  Bottom 0.152: v22.35,27.94 24.89,25.4 v24.89,25.15
POE+
  Bottom 0.61: J1.9 19.43,20.95 20.32,21.84 20.32,28.45 18.41,30.35 9.53,30.35 8.89,30.99 4.19,30.99 3.05,32.13 3.05,33.34 J15.1
POE-  (via drill 0.3 pad 0.61)
  Top 0.559: J15.2 0.64,31.21 0.64,25.91 6.86,19.68 v6.86,18.67 v7.37,18.16 v7.87,17.65
  Bottom 0.559: J1.10 19.3,15.88 9.65,15.88 v6.86,18.67
RST_N
  Top 0.152: R5.1 23.03,41.82 22.1,40.89 22.1,40.01 21.59,39.5 21.59,35.94 21.08,35.43 18.92,35.43 18.62,35.73 U1.37
RX_CAN  (via drill 0.3 pad 0.61)
  Top 0.152: U2.32 15.38,50.94 v15.49,51.05 15.49,54.1 17.14,55.75 17.14,59.56 D6.- | U4.4 v25.4,47.12
  Bottom 0.152: v15.49,51.05 15.49,52.2 16,52.7 17.78,52.7 19.43,51.05 20.95,51.05 24.89,47.12 v25.4,47.12
RXN
  Top 0.152: U1.5 12.27,32.63 12.38,32.51 13.21,32.51 13.59,32.13 13.59,29.34 12.32,28.07 12.32,27.43 10.29,25.4 8.76,25.4 8.64,25.27 8.64,25.02 9.14,24.51 C11.1
  Top 0.305: R24.1 C11.1
RXP
  Top 0.152: U1.6 12.38,32.13 12.45,32.19 13.02,32.19 13.21,32 13.21,29.46 11.94,28.19 11.94,27.56 10.16,25.78 8.64,25.78 8.26,25.4 8.26,25.02 C12.1
  Top 0.305: C12.1 R25.2
SCK  (via drill 0.3 pad 0.61)
  Top 0.152: U1.33 19.16,33.13 v19.05,33.02 | U2.2 13.88,41.56 13.21,40.89 v13.21,39.12
  Bottom 0.152: J14.3 24.89,29.84 21.72,33.02 v19.05,33.02 19.05,33.66 19.68,34.29 19.68,35.43 18.16,36.96 18.16,38.1 17.4,38.86 13.46,38.86 v13.21,39.12
SCL
  Top 0.152: U2.22 20.07,47.47 21.49,48.9 26.42,48.9 27.94,50.42 J4.4
SCS_N  (via drill 0.3 pad 0.51, 0.3 pad 0.61)
  Top 0.152: U1.32 21.45,32.63 21.84,33.02 21.84,34.67 22.29,35.12 22.29,39.18 22.86,39.75 22.86,40.39 v23.11,40.64 23.25,40.77 R5.3 | U2.29 16.88,50.66 v17.02,50.8
  Bottom 0.152: v23.11,40.64 23.24,40.64 24.51,41.91 24.51,45.21 20.19,49.53 17.53,49.53 17.14,49.91 17.14,50.67 v17.02,50.8
SDA  (via drill 0.3 pad 0.61)
  Top 0.152: U2.21 20.07,46.97 21.36,48.26 v24.77,48.26
  Bottom 0.152: v24.77,48.26 24.77,50.67 27.43,53.34 J4.3
SWCLK  (via drill 0.3 pad 0.61)
  Top 0.152: J15.4 1.91,28.96 3.62,30.67 3.62,32.96 v3.87,33.21 | U2.45 11.96,44.47 11.3,43.81 11.3,42.29 v9.65,40.64
  Bottom 0.152: v3.87,33.21 3.87,33.59 3.05,34.42 3.05,36.83 5.08,38.86 9.14,38.86 9.53,39.24 9.53,40.51 v9.65,40.64
SWDIO  (via drill 0.3 pad 0.61)
  Top 0.152: J15.5 1.91,26.8 3.94,28.83 3.94,32.26 4.32,32.64 v4.45,32.64 | U2.46 12.09,43.97 11.68,43.56 11.68,41.53 v10.16,40.01
  Bottom 0.152: v4.45,32.64 4.45,33.66 3.43,34.67 3.43,36.7 5.21,38.48 9.53,38.48 10.16,39.12 v10.16,40.01
TOCAP
  Top 0.305: U1.20 16.62,26.4 16.38,26.16 16.38,25.65 16.76,25.27 22.61,25.27 C28.2
TX_CAN  (via drill 0.3 pad 0.61)
  Top 0.152: U2.31 15.88,50.04 v16,50.16 16.13,50.29 16.13,54.23 17.53,55.63 17.53,60.83 16.89,61.47 14.61,61.47 D7.- | U4.1 v21.59,47.24
  Bottom 0.152: v16,50.16 17.02,49.15 19.68,49.15 v21.59,47.24
TXN  (via drill 0.3 pad 0.61)
  Top 0.152: J1.6 15.24,17.65 15.24,18.29 15.37,18.41 17.65,18.41 18.29,19.05 18.29,20.7 17.72,21.27 17.72,21.91 v17.91,22.1 17.91,22.48 R27.1 | v15.88,29.46 15.62,29.72 15.62,32.51 13.59,34.54 12.38,34.54 12.3,34.63 U1.1
  Bottom 0.152: v17.91,22.1 17.78,22.23 17.78,24.89 18.29,25.4 18.29,27.05 17.65,27.69 16,27.69 15.62,28.07 15.62,29.21 v15.88,29.46
TXP  (via drill 0.3 pad 0.61)
  Top 0.152: J1.5 14.35,19.69 15.24,18.8 17.53,18.8 17.91,19.18 17.91,20.57 17.34,21.14 17.34,21.91 v17.14,22.1 17.14,22.35 16.76,22.73 R30.1 | v14.99,29.46 15.24,29.72 15.24,32.38 13.4,34.23 12.38,34.23 12.28,34.13 U1.2
  Bottom 0.152: v17.14,22.1 17.4,22.35 17.4,25.02 17.91,25.53 17.91,26.92 17.53,27.3 15.88,27.3 15.24,27.94 15.24,29.21 v14.99,29.46
USB+
  Top 0.152: USB2.B6 5.98,55.49 5.84,55.63 5.84,56.2 6.1,56.45 6.86,56.45 6.98,56.33 USB2.A6 6.98,54.3 7.05,54.23 7.05,53.85 7.56,53.34 13.84,53.34 14.35,52.83 14.38,52.8 14.48,52.7 14.48,50.04 14.38,49.94 U2.34
USB-  (via drill 0.3 pad 0.61)
  Top 0.152: v7.49,55.88 7.48,55.87 USB2.B7 7.48,54.28 7.43,54.23 7.43,54.04 7.75,53.72 14.1,53.72 14.61,53.21 14.73,53.09 14.88,52.94 U2.33 | USB2.A7 6.48,55.81 v6.41,55.88
  Bottom 0.152: v6.41,55.88 v7.49,55.88
WINT_N
  Top 0.152: U1.36 21.29,34.63 21.97,35.31 21.97,39.37 22.48,39.88 22.48,40.77 22.98,41.27 R5.2
XO
  Top 0.254: U1.31 22.35,32.13 22.73,32.51 22.73,35.43 X2.2 23.62,37.85 C26.2

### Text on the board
tPlace: CANH | CANL | RST | USR | R | P | L
bPlace: 0 | 1 | Squama Ethernet with CAN FD | 2 | ANALOG | A0 | 3 | 4 | A1 | DIGITAL IO | 3V | 5 | POWER | 6 | 5V | GND | longan-labs.cc | 7 | 12/17/2020 | PoE+ | G | PoE- | 5V | 3V | V1.0 | SCK | SWCLK | SPI | MISO | SWDIO | MOSI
